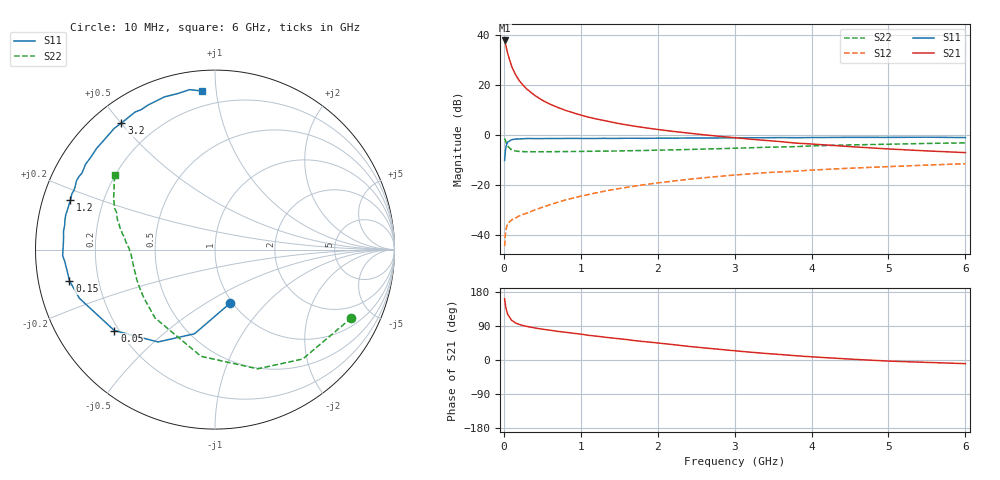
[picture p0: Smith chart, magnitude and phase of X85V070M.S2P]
! SIEMENS Small Signal Semiconductors
! BFP136W
! Si NPN RF Bipolar Junction Transistor in SOT343
! VCE = 5 V  IC = 70 mA
! Common Emitter S-Parameters:  September  1994
# GHz  S  MA  R  50
!  f  S11  S21  S12  S22
! GHz  MAG  ANG  MAG  ANG  MAG  ANG  MAG  ANG
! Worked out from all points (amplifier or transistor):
!   40 points, 10 MHz to 6 GHz, reference 50 ohm
!   highest |S21| = 37.6 dB at 10 MHz (marker M1)
!   |S21| within 3 dB of that: start of sweep to 34.05 MHz
!   unconditionally stable (mu >= 1): 618.9 MHz to 2.905 GHz
!   at 200 MHz: K = 0.60, MSG = 27.0 dB, |S12| = -32.3 dB
!   at 1.5 GHz: K = 1.11, MAG = 10.9 dB, |S12| = -21.3 dB
!   at 6 GHz: K = 0.96, MSG = 2.2 dB, |S12| = -11.5 dB
!   S11 on the Smith chart (normalised r, x): 10 MHz: 0.98, -0.64; 50 MHz: 0.18, -0.34; 150 MHz: 0.09, -0.11; 1.2 GHz: 0.08, +0.17; 3.2 GHz: 0.08, +0.50; 6 GHz: 0.11, +0.92
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0.01  0.309 -73.8  76.12 161.8  0.0061 69.6  0.8501 -26.6
0.02  0.4828 -103.7  66.6 146.4  0.0105 59.4  0.7813 -51.3
0.03  0.6047 -121.7  57.44 134.9  0.0137 50.5  0.7052 -70.4
0.05  0.7196 -141.2  41.92 120.4  0.0173 39.0  0.5994 -97.5
0.1  0.803 -160.3  23.54 105.0  0.0202 34.2  0.5065 -131.2
0.15  0.8292 -167.9  16.09 98.0  0.0221 35.1  0.4789 -146.0
0.2  0.833 -172.3  12.11 93.9  0.0244 37.2  0.47 -154.2
0.25  0.84 -175.6  9.78 90.9  0.0262 39.8  0.4665 -159.4
0.3  0.8496 -177.7  8.18 88.6  0.0278 42.5  0.4634 -162.9
0.4  0.8457 178.2  6.16 84.6  0.032 46.8  0.4632 -167.5
0.5  0.8462 175.4  4.912 81.4  0.0362 49.8  0.4635 -170.6
0.6  0.8502 173.2  4.101 78.7  0.0408 52.7  0.4641 -172.6
0.7  0.8485 170.6  3.533 75.6  0.0456 55.1  0.4656 -174.0
0.9  0.8537 166.9  2.765 70.7  0.0553 57.2  0.4678 -176.6
1.1  0.8509 162.6  2.259 65.1  0.0651 58.2  0.4721 -178.2
1.2  0.8513 161.1  2.086 63.0  0.0704 58.7  0.475 -179.0
1.7  0.8602 151.7  1.496 51.2  0.0957 57.6  0.4869 177.1
2.2  0.8623 143.3  1.177 40.6  0.1207 54.5  0.5041 173.5
3.2  0.877 126.5  0.824 20.7  0.1677 45.7  0.5543 164.9
4.5  0.8963 108.3  0.586 2.4  0.2177 33.9  0.6332 153.1
5.5  0.9023 99.0  0.481 -6.3  0.251 26.0  0.6776 146.1
6  0.8866 94.7  0.445 -9.6  0.2676 21.7  0.6946 143.0
